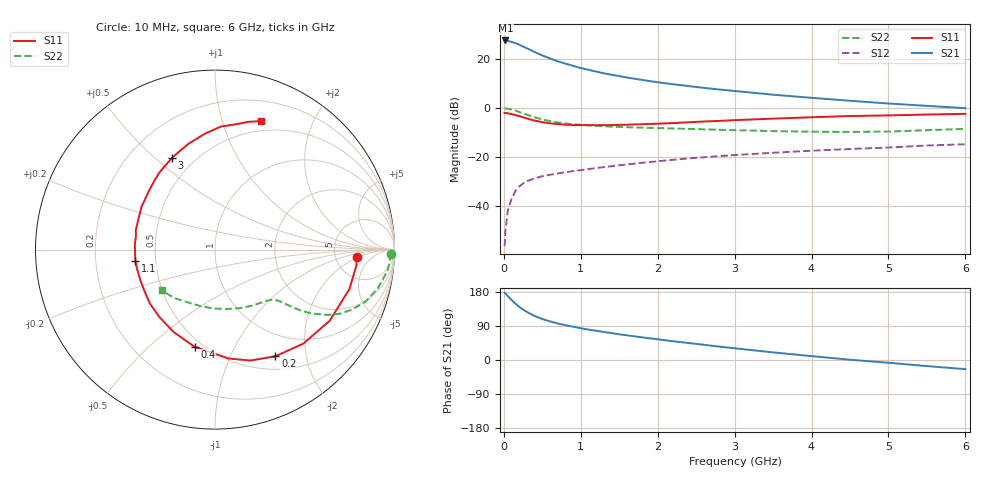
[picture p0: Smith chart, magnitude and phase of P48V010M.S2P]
! SIEMENS Small Signal Semiconductors
! BFP182
! Si NPN RF Bipolar Junction Transistor in SOT143
! VCE = 8 V  IC = 10 mA
! Common Emitter S-Parameters:  March  1996
# GHz  S  MA  R  50
!  f  S11  S21  S12  S22
! GHz  MAG  ANG  MAG  ANG  MAG  ANG  MAG  ANG
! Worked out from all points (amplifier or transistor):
!   36 points, 10 MHz to 6 GHz, reference 50 ohm
!   highest |S21| = 27.6 dB at 20 MHz (marker M1)
!   |S21| within 3 dB of that: start of sweep to 286 MHz
!   unconditionally stable (mu >= 1): 1.275 GHz to 5.611 GHz
!   at 250 MHz: K = 0.30, MSG = 28.0 dB, |S12| = -30.9 dB
!   at 1.4 GHz: K = 1.04, MAG = 17.5 dB, |S12| = -23.8 dB
!   at 6 GHz: K = 0.96, MSG = 7.4 dB, |S12| = -14.8 dB
!   lowest NFmin = 1.50 dB at 450 MHz
!   S11 on the Smith chart (normalised r, x): 10 MHz: 8.14, -1.79; 200 MHz: 0.67, -1.50; 400 MHz: 0.45, -0.71; 1.1 GHz: 0.38, -0.06; 3 GHz: 0.38, +0.57; 6 GHz: 0.40, +1.35
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0.01  0.7904 -3.0  23.94 177.2  0.0015 84.5  0.9812 -1.3
0.02  0.7927 -6.5  24.07 175.5  0.003 82.7  0.9782 -2.7
0.05  0.7806 -16.3  23.76 168.8  0.0077 83.1  0.9685 -7.0
0.1  0.7523 -31.8  22.48 158.5  0.0139 73.5  0.9319 -13.5
0.15  0.7188 -46.8  21.3 148.7  0.0201 66.6  0.8859 -19.2
0.2  0.683 -60.5  19.75 140.3  0.0249 62.8  0.8316 -23.8
0.25  0.6488 -72.3  18.05 133.0  0.0286 57.6  0.7803 -27.3
0.3  0.6114 -82.9  16.66 126.9  0.0321 54.3  0.7286 -30.0
0.4  0.5533 -101.9  14 116.2  0.0364 49.5  0.6456 -33.5
0.5  0.5141 -116.6  11.85 108.2  0.0404 46.8  0.5857 -35.4
0.6  0.4872 -129.4  10.35 101.9  0.0432 45.0  0.5426 -36.5
0.7  0.4711 -140.3  9.035 96.5  0.046 44.6  0.5093 -37.3
0.9  0.4496 -157.5  7.288 87.9  0.0512 43.9  0.4657 -38.3
1.1  0.4481 -172.2  6.052 80.2  0.0566 44.0  0.4414 -39.7
1.3  0.4476 176.3  5.136 73.9  0.062 43.7  0.4239 -41.3
1.6  0.4563 161.3  4.22 65.1  0.0703 43.8  0.4061 -44.5
2.2  0.493 138.2  3.062 49.5  0.0873 41.7  0.3821 -52.9
3  0.5651 115.1  2.231 30.9  0.1094 36.8  0.3526 -67.8
3.5  0.6071 104.2  1.875 20.1  0.1218 33.0  0.3372 -78.9
4.5  0.6862 87.3  1.407 0.7  0.1454 25.7  0.3249 -104.2
5.5  0.7364 75.2  1.108 -16.1  0.1714 18.8  0.3525 -130.2
6  0.7613 70.2  0.994 -24.1  0.1818 14.3  0.3747 -142.6
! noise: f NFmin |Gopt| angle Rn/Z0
0.45  1.5  0.26  43  0.28
0.9  1.6  0.24  87  0.22
1.8  2.1  0.2  170  0.2
